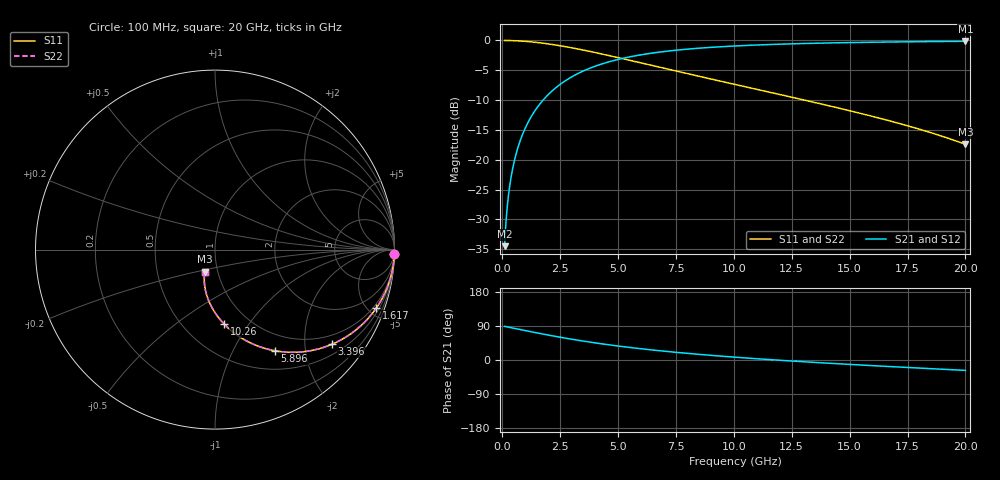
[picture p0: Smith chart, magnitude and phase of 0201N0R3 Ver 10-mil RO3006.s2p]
# GHz S MA R 50
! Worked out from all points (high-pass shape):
!   1601 points, 100 MHz to 20 GHz, reference 50 ohm
!   highest |S21| = -0.14 dB at 20 GHz (marker M1); lowest = -34.5 dB at 100 MHz (marker M2)
!   |S21| within 3 dB of the highest: 5.041 GHz to end of sweep
!   lowest |S11| = -17.4 dB at 20 GHz (marker M3), VSWR 1.31, Z = 43.5 - j10.9 ohm
!   |S11| at or under -10 dB: 13.05 GHz to end of sweep
!   |S22| runs from -17.4 to 0.0 dB; largest |S21 - S12| = 0
!   S11 on the Smith chart (normalised r, x): 100 MHz: 1, -91; 1.617 GHz: 0.74, -5.60; 3.396 GHz: 0.74, -2.64; 5.896 GHz: 0.75, -1.48; 10.26 GHz: 0.77, -0.78; 20 GHz: 0.87, -0.22
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0.1  0.9998 -1.3  0.01888 88.7  0.01888 88.7  0.9998 -1.3
0.1621875  0.9995 -2.0  0.03061 87.9  0.03061 87.9  0.9995 -2.0
0.24925  0.9989 -3.1  0.04702 86.9  0.04702 86.9  0.9989 -3.1
0.323875  0.9981 -4.1  0.06105 85.9  0.06105 85.9  0.9981 -4.1
0.44825  0.9964 -5.6  0.08436 84.3  0.08436 84.3  0.9964 -5.6
0.5975  0.9936 -7.5  0.1122 82.5  0.1122 82.5  0.9936 -7.5
0.7840625  0.9891 -9.8  0.1465 80.1  0.1465 80.1  0.9891 -9.8
1.020375  0.9818 -12.7  0.1894 77.2  0.1894 77.2  0.9818 -12.7
1.294  0.9712 -16.1  0.2377 73.9  0.2377 73.9  0.9712 -16.1
1.617375  0.9559 -19.9  0.2926 70.0  0.2926 70.0  0.9559 -19.9
2.400937  0.9094 -28.8  0.4144 61.1  0.4144 61.1  0.9094 -28.8
3.395938  0.8383 -39.0  0.5431 50.9  0.5431 50.9  0.8383 -39.0
3.420812  0.8364 -39.2  0.546 50.6  0.546 50.6  0.8364 -39.2
4.540188  0.7518 -49.2  0.6566 40.6  0.6566 40.6  0.7518 -49.2
5.895875  0.6547 -59.4  0.7525 30.3  0.7525 30.3  0.6547 -59.4
6.741625  0.5997 -64.9  0.7965 24.8  0.7965 24.8  0.5997 -64.9
8.30875  0.5103 -73.7  0.8557 15.8  0.8557 15.8  0.5103 -73.7
10.05  0.4278 -82.0  0.899 7.4  0.899 7.4  0.4278 -82.0
10.26144  0.4188 -82.9  0.9032 6.5  0.9032 6.5  0.4188 -82.9
13.37081  0.3061 -94.9  0.9462 -5.9  0.9462 -5.9  0.3061 -94.9
16.69162  0.2129 -105.5  0.9705 -17.2  0.9705 -17.2  0.2129 -105.5
20  0.1347 -114.5  0.9835 -27.4  0.9835 -27.4  0.1347 -114.5
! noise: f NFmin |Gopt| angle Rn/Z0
0.1  0.001509  0.9819  0.9985  0.01897
2.301  0.005471  0.836  6.344  0.00703
4.515  0.008345  0.7894  9.995  0.0081
6.729  0.01084  0.7608  13.7  0.009056
8.943  0.01312  0.7403  17.43  0.009897
11.14  0.01526  0.7247  21.12  0.01065
13.36  0.01732  0.7124  24.82  0.01134
15.57  0.01933  0.7025  28.48  0.01199
17.79  0.02129  0.6946  32.1  0.01259
20  0.02322  0.6883  35.68  0.01317
